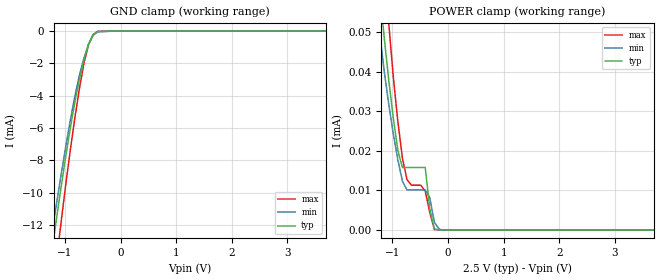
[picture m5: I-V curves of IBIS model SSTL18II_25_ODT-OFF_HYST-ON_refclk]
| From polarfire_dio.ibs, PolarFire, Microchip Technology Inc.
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|   Model SSTL18II_25_ODT-OFF_HYST-ON_refclk
[Model]   SSTL18II_25_ODT-OFF_HYST-ON_refclk
Model_type   Input
Vinl =   0.775
Vinh =   1.025
|   typ   min   max
C_comp   5.210e-12   5.210e-12   5.520e-12
[Temperature Range]  25C   100C   -40C
[Voltage Range]  2.5   2.375   2.625
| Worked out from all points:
|   GND clamp passes 1 mA (typ) near -0.59 V on its own axis
[GND Clamp]
| Voltage   I(typ)   I(min)   I(max)
-2.5V     -50.62mA   -47.15mA   -57.43mA
-1.23V    -13.52mA   -12.43mA   -16.52mA
-1.148V   -11.52mA   -10.6mA    -14.11mA
-1.066V   -9.581mA   -8.827mA   -11.74mA
-902.3mV  -5.975mA   -5.502mA   -7.338mA
-820.3mV  -4.378mA   -4.012mA   -5.35mA
-738.3mV  -2.961mA   -2.707mA   -3.528mA
-656.2mV  -1.735mA   -1.644mA   -1.964mA
-574.2mV  -787.2uA   -824.8uA   -813.2uA
-492.2mV  -214.7uA   -270uA     -208.1uA
-410.2mV  -22.22uA   -41.6uA    -20.31uA
5V        0A         0A         0A
[POWER Clamp]
| Voltage   I(typ)   I(min)   I(max)
-2.5V     316.7uA    224.8uA    405.4uA
-1.312V   73.32uA    59.52uA    99.49uA
-1.148V   48.63uA    40.16uA    66.69uA
-1.066V   37.84uA    31.74uA    52.11uA
-902.3mV  20.05uA    17.67uA    27.31uA
-820.3mV  15.78uA    12.33uA    18.14uA
-738.3mV  15.78uA    10.1uA     12.71uA
-410.2mV  15.78uA    10.1uA     9.821uA
-328.1mV  5.283uA    8.134uA    4.392uA
-246.1mV  272.4nA    1.951uA    116nA
-82.03mV  9.588nA    24.05nA    13.02nA
5V        0A         0A         0A
